// TwinCAT 3 PLC project Novram_Test
// ProgramVersion: 3.1.4023.0
// libraries:
//   Tc2_IoFunctions, * (Beckhoff Automation GmbH)
//   Tc2_Standard, * (Beckhoff Automation GmbH)
//   Tc2_System, * (Beckhoff Automation GmbH)
//   Tc3_Module, * (Beckhoff Automation GmbH)
// project tree:
//   DUTs/ DUT_Novram_Struct.TcDUT
//   / PlcTask.TcTTO
//   POUs/ MAIN.TcPOU
// real-time tasks:
//   TASK PlcTask: cycle T#10ms, priority 21, ADS port 350
// I/O:
//   DEVICE Device 4 (NOV-DP-RAM)
//     Box 1 (Retain Handler)
// variable links:
//   Novram Test/Novram Test Instance <-> Device 4 (NOV-DP-RAM)/Box 1 (Retain Handler)
//     PlcTask Retains/MAIN.ST_Novram1.f_height <-> Retains/MAIN.ST_Novram1.f_height_[0]
//     PlcTask Retains/MAIN.ST_Novram1.f_height <-> Retains/MAIN.ST_Novram1.f_height_[851]
//     PlcTask Retains/MAIN.ST_Novram1.f_weight <-> Retains/MAIN.ST_Novram1.f_weight_[0]
//     PlcTask Retains/MAIN.ST_Novram1.f_weight <-> Retains/MAIN.ST_Novram1.f_weight_[851]
//     PlcTask Retains/MAIN.ST_Novram1.i_old <-> Retains/MAIN.ST_Novram1.i_old_[0]
//     PlcTask Retains/MAIN.ST_Novram1.i_old <-> Retains/MAIN.ST_Novram1.i_old_[851]
//     PlcTask Retains/MAIN.ST_Novram1.s_gender <-> Retains/MAIN.ST_Novram1.s_gender_[0]
//     PlcTask Retains/MAIN.ST_Novram1.s_gender <-> Retains/MAIN.ST_Novram1.s_gender_[851]
//     PlcTask Retains/MAIN.ST_Novram1.s_name <-> Retains/MAIN.ST_Novram1.s_name_[0]
//     PlcTask Retains/MAIN.ST_Novram1.s_name <-> Retains/MAIN.ST_Novram1.s_name_[851]
//     PlcTask Retains/MAIN.ST_Novram2 <-> Retains/MAIN.ST_Novram2_[0]
//     PlcTask Retains/MAIN.ST_Novram2 <-> Retains/MAIN.ST_Novram2_[851]
//     PlcTask Retains/MAIN.arr_Array <-> Retains/MAIN.arr_Array_[0]
//     PlcTask Retains/MAIN.arr_Array <-> Retains/MAIN.arr_Array_[851]
//     PlcTask Retains/MAIN.b_bool <-> Retains/MAIN.b_bool_[0]
//     PlcTask Retains/MAIN.b_bool <-> Retains/MAIN.b_bool_[851]
//     PlcTask Retains/MAIN.f_real <-> Retains/MAIN.f_real_[0]
//     PlcTask Retains/MAIN.f_real <-> Retains/MAIN.f_real_[851]
//     PlcTask Retains/MAIN.i_int <-> Retains/MAIN.i_int_[0]
//     PlcTask Retains/MAIN.i_int <-> Retains/MAIN.i_int_[851]

CONFIGURATION Novram_Test
    RESOURCE PLC ON TwinCAT3
        TASK PlcTask(INTERVAL := T#10ms, PRIORITY := 21);
        PROGRAM MAIN WITH PlcTask : MAIN;
    END_RESOURCE
END_CONFIGURATION

// ---- DUTs/DUT_Novram_Struct.TcDUT
TYPE DUT_Novram_Struct :
STRUCT RETAIN
	s_name: WSTRING;
	i_old: INT;
	s_gender: WSTRING;
	f_height: LREAL;
	f_weight: LREAL;
END_STRUCT
END_TYPE

// ---- POUs/MAIN.TcPOU
PROGRAM MAIN
VAR
	ST_Novram1: DUT_Novram_Struct;
END_VAR

VAR RETAIN
	b_bool: BOOL;
	i_int: INT;
	f_real: REAL;
	arr_Array: ARRAY[0..1023] OF byte;
	ST_Novram2: DUT_GVL_Novram_Struct;
END_VAR

END_PROGRAM
